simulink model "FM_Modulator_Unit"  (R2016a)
settings: Solver=ode3  StartTime=0.0  StopTime=1  FixedStep=1/5000000  RelTol=1e-3

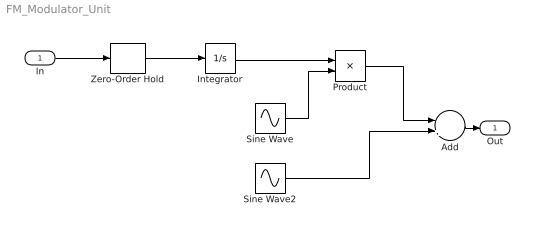
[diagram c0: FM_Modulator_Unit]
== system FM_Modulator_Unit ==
  In : Inport
  Add : Sum  Inputs=-+
  Integrator : Integrator
  Product : Product
  Sine Wave : Sin  Frequency=500000*2*pi  Phase=-0.5*pi
  Sine Wave2 : Sin  Frequency=500000*2*pi
  Zero-Order Hold : ZeroOrderHold  SampleTime=1/5000000
  Out : Outport
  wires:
  Zero-Order Hold/1 -> Integrator/1
  In/1 -> Zero-Order Hold/1
  Sine Wave/1 -> Product/2
  Sine Wave2/1 -> Add/2
  Product/1 -> Add/1
  Integrator/1 -> Product/1
  Add/1 -> Out/1
